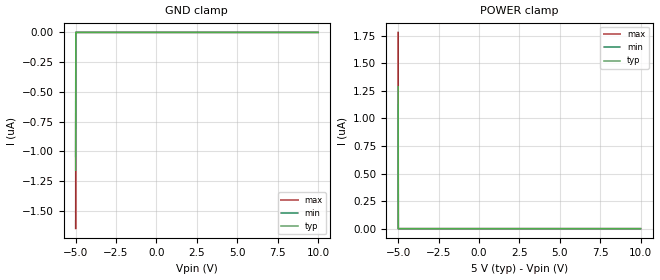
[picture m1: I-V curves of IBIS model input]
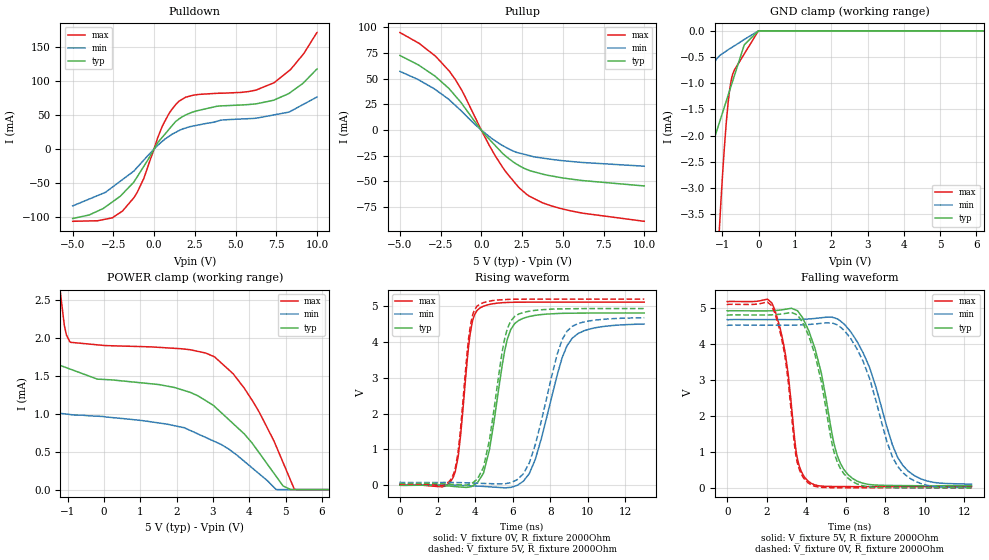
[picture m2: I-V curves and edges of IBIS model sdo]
|Texas Instruments Incorporated
| 16-Bit, Single Channel, Digital-to-Analog Converter W/ Internal +10V
| Reference and Serial I/F
| Marketing part#   Digital Voltage Range   Package-type   #pins
| DAC7731E   4.75V - 5.25V   SSOP   24
| DAC7731E/1K   4.75V - 5.25V   SSOP   24
| DAC7731E/1KG4   4.75V - 5.25V   SSOP   24
| DAC7731EB   4.75V - 5.25V   SSOP   24
| DAC7731EB/1K   4.75V - 5.25V   SSOP   24
| DAC7731EB/1KG4   4.75V - 5.25V   SSOP   24
| DAC7731EBG4   4.75V - 5.25V   SSOP   24
| DAC7731EC   4.75V - 5.25V   SSOP   24
| DAC7731EC/1K   4.75V - 5.25V   SSOP   24
| DAC7731EC/1KG4   4.75V - 5.25V   SSOP   24
| DAC7731ECG4   4.75V - 5.25V   SSOP   24
| DAC7731EG4   4.75V - 5.25V   SSOP   24
[IBIS Ver]   3.2
[File name]   dac7731.ibs
[File Rev]   1.0
[Date]   12/ 9/ 2011
[Source]
| Texas Instruments Incorporated.
| Analog-eLab Design Center, HPA
| 12500 TI Blvd
| Dallas, TX -75243
| e-mail: elab_scm_ibis@list.ti.com
[Notes]   Revision History:
| Rev 1.0: 12/9/2011
| - Initial version of the model
| - Model generated from simulations in SPECTRE
| - Model matched to SPICE simulation
| - C_comp although listed in numerical order of value are
|   obtained from varying PVT conditions. For PVT conditions for
|   each specific value refer the buffer description under
|   respective [Model]. IBIS model user is responsible for using
|   appropriate C_comp to simulate for Signal Integrity.
|*  EXCEPTION:   *
|*  - For model sdo, there will be a leakage current in the POWER   *
|*   clamp I-V table because of the transistor(n2) connected to the pad*
[Disclaimer]
| This model is designed as an aid for customers of Texas Instruments.
| TI and its licensors and suppliers make no warranties, either expressed
| or implied, with respect to this  model, including the warranties of
| merchantability or fitness for a particular purpose. The model is
| provided solely on an "as is" basis. The entire risk as to its quality
| and performance is with the customer.
[Copyright]
 (C) Copyright 2011 Texas Instruments Incorporated.All rights reserved.
|   DAC7731
[Component]   DAC7731
[Manufacturer]   TI
[Package]   |24 SSOP  -  DB package
|   typ   min   max
R_pkg   0.10158   0.05230   0.14184
L_pkg   2.49967nH   1.93186nH   2.98186nH
C_pkg   0.40655pF   0.36455pF   0.54145pF
[Pin]  signal_name   model_name   R_pin   L_pin   C_pin
1   VCC   power   0.10027   3.48965nH  0.51968pF
2   REFOUT   term   0.05457   2.65799nH  0.54145pF
3   REFIN   term   0.12059   2.63947nH  0.39045pF
4   REFADJ   term   0.05230   1.93186nH  0.40053pF
5   VREF   term   0.09888   2.26060nH  0.36510pF
6   ROFFSET   term   0.09827   2.25170nH  0.36455pF
7   AGND   gnd   0.09882   2.26070nH  0.36641pF
8   RFB2   term   0.10701   2.37858nH  0.37267pF
9   RFB1   term   0.12064   2.57687nH  0.38178pF
10   SJ   term   0.14184   2.95497nH  0.40274pF
11   VOUT   term   0.10246   2.98186nH  0.50316pF
12   VDD   power   0.09531   3.42256nH  0.52399pF
13   DGND   gnd   0.09530   3.42234nH  0.52342pF
14   TEST   term   0.09897   2.93263nH  0.50071pF
15   NC   NC   0.11223   2.52302nH  0.38216pF
16   _RST   input   0.11508   2.49656nH  0.37533pF
17   LDAC   input   0.10327   2.32513nH  0.36959pF
18   SDI   input   0.09759   2.24326nH  0.36537pF
19   SDO   sdo   0.10014   2.27796nH  0.36565pF
20   _CS   input   0.10143   2.29654nH  0.36589pF
21   SCLK   input   0.10709   2.37802nH  0.37023pF
22   RSTSEL   rst_ref   0.11979   2.62680nH  0.38857pF
23   _REFEN   rst_ref   0.08857   2.78322nH  0.49406pF
24   VSS   power   0.08939   3.33810nH  0.51126pF
|   rst_ref Model
[Model]   rst_ref
Model_type   Input
Vinl = 1.5
Vinh = 3.5
|   typ   min   max
|   (nom PVT)   (fast PVT)   (slow PVT)
|C_comp from frequency sweep method (F=20MHz)
|Average
C_comp   6.430e-14   5.528e-14   6.550e-14
|C_comp from LC tank measurement(L=1nH)
|Average
|Resonant Frequency(Hz)   1.000e+12   1.000e+12   1.000e+12
|C_comp   2.536e-17   2.536e-17   2.536e-17
| Where nom  PVT is Nominal Process, 5V, 32C
|   Fast PVT is Strong Process,  5.25V, -40C
|   Slow PVT is Weak Process,   4.75V, 92C
[Model Spec]
|Subparameter   typ   min   max
Vinh   3.5   3.325   3.675
Vinl   1.5   1.425   1.575
[Voltage Range]   5   4.75   5.25
|Ambient Temperature   25   85   -40
|Junction Temperature
[Temperature Range]   32   92   -40
[Power Clamp Reference]   5   4.75   5.25
[GND Clamp Reference]   0   0   0
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[Model] term
Model_type Terminator
C_comp   1.0e-20F  1.0e-20F  1.0e-20F
|   typ   min   max
[Voltage Range]   5.0V   4.75V   5.25V
[POWER Clamp Reference]   5.0V   4.75V   5.25V
[GND Clamp Reference]   0V   0V   0V
|Ambient Temperature   25   85   -40
|Junction Temperature
[Temperature Range]   32   92   -40
| Models and submodels in the file (4): input (Input), rst_ref (Input), sdo (3-state), term (Terminator)
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|   input Model
[Model]   input
Model_type   Input
Vinl = 1.5
Vinh = 3.5
|   typ   min   max
|   (nom PVT)   (fast PVT)   (slow PVT)
|C_comp from frequency sweep method (F=20MHz)
|Average
C_comp   1.742e-13   1.711e-13   1.772e-13
|C_comp from LC tank measurement(L=1nH)
|Average
|Resonant Frequency(Hz)   1.000e+12   1.000e+12   1.000e+12
|C_comp   2.536e-17   2.536e-17   2.536e-17
| Where nom  PVT is Nominal Process, 5V, 32C
|   Fast PVT is Strong Process,  5.25V, -40C
|   Slow PVT is Weak Process,   4.75V, 92C
[Model Spec]
|Subparameter   typ   min   max
Vinh   3.5   3.325   3.675
Vinl   1.5   1.425   1.575
[Voltage Range]   5   4.75   5.25
|Ambient Temperature   25   85   -40
|Junction Temperature
[Temperature Range]   32   92   -40
[Power Clamp Reference]   5   4.75   5.25
[GND Clamp Reference]   0   0   0
[GND Clamp]
|   Voltage   I(typ)   I(min)   I(max)
-5V       -1.16uA    -1.043uA   -1.65uA
-4.99V    -58.02nA   0A         -157.2nA
-4.99V    0A         0A         -78.58nA
-4.989V   0A         0A         0A
10V       0A         0A         0A
[POWER Clamp]
|   Voltage   I(typ)   I(min)   I(max)
-5V       1.291uA    1.125uA    1.782uA
-4.99V    64.53nA    0A         169.7nA
-4.99V    0A         0A         84.84nA
-4.989V   0A         0A         0A
10V       0A         0A         0A
|   sdo Model
[Model]   sdo
Model_type   3-state
Polarity   Non-Inverting
Vmeas = 2.5
Vref = 2.5
Cref = 200pF
Rref = 2000
|   typ   min   max
|   (nom PVT)   (fast PVT)   (slow PVT)
|C_comp from frequency sweep method (F=10MHz)
C_comp   4.265e-12   3.993e-12   4.520e-12
|ON state : BUFFER OUTPUT TURNED HIGH
|C_comp   4.265e-12   3.993e-12   4.520e-12
|OFF state: BUFFER OUTPUT TURNED LOW
|C_comp   2.275e-12   2.294e-12   2.252e-12
|C_comp from LC tank measurement(L=1nH)
|Resonant Frequency(Hz)   3.660e+09   3.680e+09   3.610e+09
|C_comp   1.893e-12   1.872e-12   1.946e-12
|ON state : BUFFER OUTPUT TURNED HIGH
|Resonant Frequency(Hz)   3.660e+09   3.680e+09   3.610e+09
|C_comp   1.893e-12   1.872e-12   1.946e-12
|OFF state: BUFFER OUTPUT TURNED LOW
|Resonant Frequency(Hz)   3.660e+09   3.680e+09   3.610e+09
|C_comp   1.893e-12   1.872e-12   1.946e-12
| Where nom  PVT is Nominal Process, 5V, 32C
|   Fast PVT is Strong Process,  5.25V, -40C
|   Slow PVT is Weak Process,   4.75V, 92C
[Voltage Range]   5   4.75   5.25
|Ambient Temperature   25   85   -40
|Junction Temperature
[Temperature Range]   32   92   -40
[Pullup Reference]   5   4.75   5.25
[Pulldown Reference]   0   0   0
[Power Clamp Reference]   5   4.75   5.25
[GND Clamp Reference]   0   0   0
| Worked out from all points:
|   slope of the pulldown table from 0 to 0.75 V, typ, clamps not added: 30.8 ohm
|   slope of the pullup table from 0 to 0.75 V, typ, clamps not added: 56 ohm
|   GND clamp passes 1 mA (typ) near -0.73 V on its own axis
|   falling waveform, V_fixture 5V, R_fixture 2000Ohm: 20-80 % time 1.11ns typ, 1.62ns min, 684ps max; typ from 4.93 V to 0.059 V
|   rising waveform, V_fixture 0V, R_fixture 2000Ohm: 20-80 % time 866ps typ, 1.36ns min, 556ps max; typ from 0 V to 4.8 V
|   rising waveform, V_fixture 5V, R_fixture 2000Ohm: 20-80 % time 859ps typ, 1.31ns min, 547ps max; typ from 0.051 V to 4.93 V
|   falling waveform, V_fixture 0V, R_fixture 2000Ohm: 20-80 % time 1.07ns typ, 1.54ns min, 668ps max; typ from 4.82 V to 0.001 V
[Pulldown]
|   Voltage   I(typ)   I(min)   I(max)
-5V       -101.9mA   -83.39mA   -105.9mA
-3.125V   -87.19mA   -64.81mA   -103.5mA
-1.944V   -65.91mA   -44.81mA   -91.02mA
-1.036V   -40.6mA    -26.8mA    -63.49mA
-626.8mV  -25.14mA   -16mA      -42.75mA
554.5mV   18.79mA    12.37mA    35.99mA
1.542V    44.37mA    27.24mA    70.42mA
3.865V    62.82mA    40.81mA    81.82mA
5.778V    65.33mA    44.6mA     84.29mA
7.369V    71.97mA    50.18mA    97.37mA
8.393V    83.53mA    55.65mA    117mA
10V       117.4mA    76.28mA    170.9mA
[GND Clamp]
|   Voltage   I(typ)   I(min)   I(max)
-5V       -67.36mA   -50.02mA   -81.31mA
-1.835V   -8.7mA     -4.113mA   -16.38mA
-1.724V   -7.292mA   -3.271mA   -14.22mA
-1.525V   -4.769mA   -1.836mA   -10.83mA
-1.25V    -2.119mA   -681.6uA   -6.144mA
-1.11V    -1.815mA   -501.3uA   -4.158mA
-1.062V   -1.713mA   -466.2uA   -3.557mA
-842mV    -1.235mA   -362.7uA   -1.387mA
-737mV    -1.008mA   -316.8uA   -886.9uA
-395mV    -266.5uA   -164.6uA   -440.6uA
-5mV      -70.85nA   -840nA     -2.229uA
10V       0A         0A         0A
[Pullup]
|   Voltage   I(typ)   I(min)   I(max)
-5V       72.73mA    57.22mA    95.06mA
-3.824V   63.07mA    48.7mA     84.56mA
-2.816V   52.18mA    39.37mA    72.03mA
-1.966V   40.07mA    29.42mA    57.38mA
-1.241V   26.67mA    18.83mA    39.88mA
30mV      -706.4uA   -454.5uA   -1.123mA
880mV     -15.59mA   -10.79mA   -25.79mA
1.515V    -25.65mA   -16.91mA   -41.06mA
2.796V    -38.47mA   -24.31mA   -62.81mA
3.862V    -43.35mA   -27.54mA   -71.5mA
5.353V    -47.45mA   -30.36mA   -78.28mA
10V       -54.46mA   -35.2mA    -88.92mA
[POWER Clamp]
|   Voltage   I(typ)   I(min)   I(max)
-5V       49.17mA    34.7mA     75.19mA
-1.918V   4.92mA     2.815mA    9.236mA
-1.577V   2.785mA    1.897mA    5.269mA
-1.248V   1.649mA    1.011mA    2.792mA
-1.036V   1.611mA    998.2uA    2.045mA
-915.5mV  1.59mA     991.2uA    1.946mA
1.945V    1.349mA    843.9uA    1.867mA
3.048V    1.097mA    635.3uA    1.752mA
4.13V     581.1uA    266.4uA    1.142mA
4.747V    170.5uA    0A         566.4uA
5.243V    0A         0A         2.491uA
10V       0A         0A         0A
[Ramp]
R_load = 2000
|   typ   min   max
dV/dt_r   2.88315/8.66355e-10   2.70659/1.37049e-09   3.06413/5.5636e-10
dV/dt_f   2.92569/1.10801e-09   2.75719/1.62871e-09   3.09583/6.83981e-10
[Falling Waveform]
V_fixture = 5V
V_fixture_min = 4.75V
V_fixture_max = 5.25V
R_fixture = 2000Ohm
|   Time   V(typ)   V(min)   V(max)
0s        4.934V     4.689V     5.193V
2.257ns   4.935V     4.688V     5.154V
2.947ns   4.977V     4.687V     3.715V
3.545ns   4.939V     4.69V      835.2mV
4.098ns   4.412V     4.705V     187.5mV
5.451ns   1.127V     4.73V      37.89mV
6.115ns   369.5mV    4.438V     36.03mV
7.205ns   93.41mV    3.352V     33.97mV
8.893ns   64.43mV    622.3mV    33.54mV
12.37ns   59.36mV    103.8mV    33.49mV
[Rising Waveform]
V_fixture = 0V
V_fixture_min = 0V
V_fixture_max = 0V
R_fixture = 2000Ohm
|   Time   V(typ)   V(min)   V(max)
0s        169.8pV    269.2pV    102.8pV
2.858ns   -32.69mV   1.179mV    251.7mV
3.097ns   -44.13mV   -942.6uV   786.8mV
3.741ns   -41.71mV   -15.13mV   4.235V
4.255ns   178.8mV    -26.46mV   4.942V
5.578ns   3.758V     -71.68mV   5.094V
6.115ns   4.512V     -24.3mV    5.103V
7.205ns   4.738V     723.1mV    5.106V
9.169ns   4.797V     4.099V     5.106V
13.01ns   4.804V     4.497V     5.107V
[Rising Waveform]
V_fixture = 5V
V_fixture_min = 4.75V
V_fixture_max = 5.25V
R_fixture = 2000Ohm
|   Time   V(typ)   V(min)   V(max)
0s        51.02mV    76.89mV    31.49mV
2.813ns   23.31mV    77.54mV    266mV
3.097ns   14.01mV    74.26mV    931mV
3.741ns   33.85mV    64.31mV    4.424V
4.098ns   162.8mV    57.82mV    4.991V
5.578ns   4.094V     42.16mV    5.177V
6.115ns   4.712V     124.3mV    5.187V
6.885ns   4.853V     621.3mV    5.189V
8.893ns   4.921V     4.296V     5.19V
13.01ns   4.928V     4.672V     5.19V
[Falling Waveform]
V_fixture = 0V
V_fixture_min = 0V
V_fixture_max = 0V
R_fixture = 2000Ohm
|   Time   V(typ)   V(min)   V(max)
0s        4.819V     4.534V     5.114V
2.257ns   4.821V     4.532V     5.072V
2.947ns   4.861V     4.531V     3.574V
3.526ns   4.823V     4.536V     754.6mV
4.098ns   4.27V      4.552V     139.1mV
5.451ns   908.6mV    4.566V     3.877mV
6.115ns   269.4mV    4.254V     3.07mV
6.885ns   57.63mV    3.516V     2.831mV
8.632ns   6.649mV    593.4mV    2.289mV
12.37ns   1.202mV    7.924mV    1.13mV
